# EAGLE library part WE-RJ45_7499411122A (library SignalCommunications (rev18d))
Order Code 7499411122A Design THT xBase-T 10/100 Base-T Ports 1x1 Application PoE+ HPLE Tab Position Up LED (Left-Right) YELLOW-GREEN EMI Fingers YES Details see: http://katalog.we-online.de/en/pbs/WE-LAN_RJ45/7499411122A? Updated by Yingchun Shan 2016-08-30 2016(C) Würth Elektronik
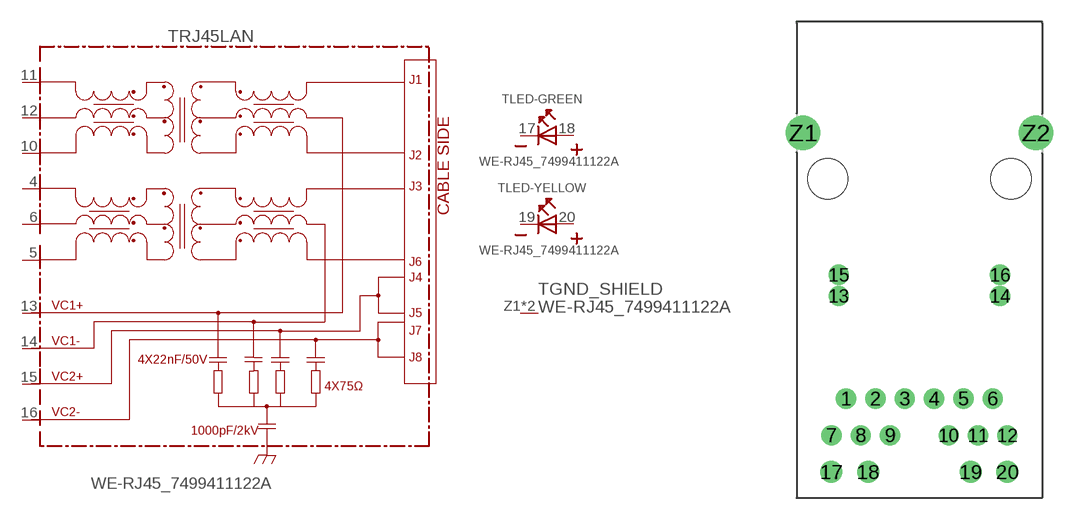
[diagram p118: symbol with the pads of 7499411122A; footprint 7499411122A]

Designator prefix T; gates RJ45LAN=7499411122A LED-GREEN=LED-2PIN LED-YELLOW=LED-2PIN GND_SHIELD=GND_PIN

## WE-RJ45_7499411122A (COMPANY-URL: http://www.we-online.de; CREATED-BY: Christin Zierenner; CREATED-DATE: AUG 2012; DATASHEET-URL: http://katalog.we-online.de/kataloge/eisos/media/pdf/7499411122A.pdf; MANUFACTURER: Würth Elektronik eiSos GmbH)  [7499411122A]
4  RJ45LAN:4
5  RJ45LAN:5
6  RJ45LAN:6
10  RJ45LAN:10
11  RJ45LAN:11
12  RJ45LAN:12
13  RJ45LAN:VC1+  pwr
14  RJ45LAN:VC1-  pwr
15  RJ45LAN:VC2+  pwr
16  RJ45LAN:VC2-  pwr
17  LED-GREEN:K  pas
18  LED-GREEN:A  pas
19  LED-YELLOW:K  pas
20  LED-YELLOW:A  pas
Z1  GND_SHIELD:1  pwr
Z2  GND_SHIELD:1  pwr

## Footprint 7499411122A (pad centres in mm)
MAX HEIGHT=13.87mm PORTS----1X1 LED --YES
drill 0.9: 1 -5.075,-15.24; 2 -3.045,-15.24; 3 -1.015,-15.24; 4 1.015,-15.24; 5 3.045,-15.24; 6 5.075,-15.24; 7 -6.09,-17.78; 8 -4.06,-17.78; 9 -2.03,-17.78; 10 2.03,-17.78; 11 4.06,-17.78; 12 6.09,-17.78
drill 0.9 pad 1.27: 13 -5.59,-8.12; 14 5.59,-8.12; 15 -5.59,-6.66; 16 5.59,-6.66
drill 1.02: 17 -6.095,-20.32; 18 -3.555,-20.32; 19 3.555,-20.32; 20 6.095,-20.32
drill 1.6: Z1 -8.065,3.18; Z2 8.065,3.18
hole 2.8 at -6.35,0
hole 2.8 at 6.35,0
